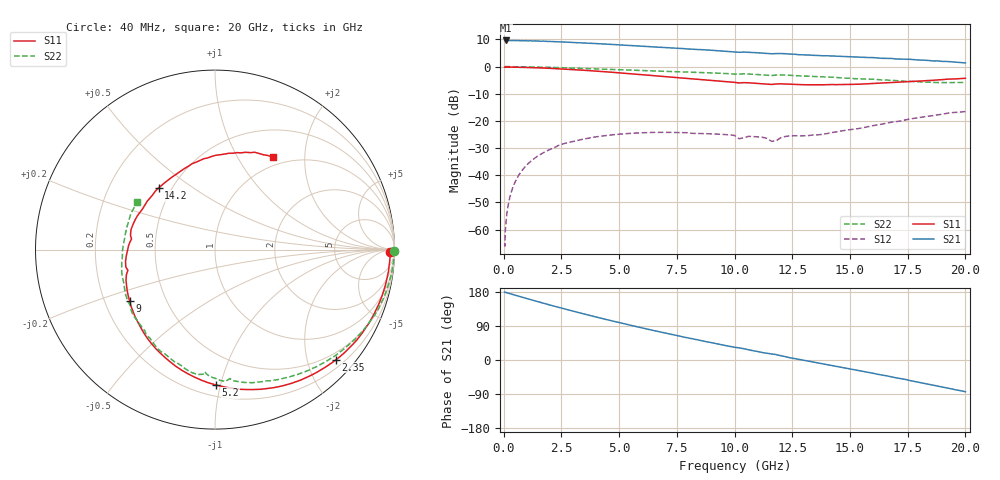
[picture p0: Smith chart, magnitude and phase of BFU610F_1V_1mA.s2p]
! Filename:  P:\Prog\Test\Noise\ATS_data\Testdata_Net\SplitFiles\BFU610_2W_A5_HighFreq_1V_1mA_D.s2p
! Date/Time: Wed 10/Aug/2011 16:54:31
! BFU610_2W_A5_HighFreq_1V_1mA_10mA_Bias1_R.s2p
! MDIF S-parameter v. bias file
! BFU610_2W_A5_HighFreq_1V_1mA_10mA
! Date/time Mon Aug 08 13:53:02 2011
! bias mode 1
! bias variable = I_out
! VAR bias_var= 1
! VAR V_out= 1.0002
! VAR I_out= 0.9900
! VAR V_in= 0.8512
! VAR I_in= 0.0075
! Device data file deembeded for feedlines and parallel
! Original file: \SplitFiles\BFU610_2W_A5_HighFreq_1V_1mA_R.s2p
! Feed-files: PR003V01_101208_Feed1.s2p, PR003V01_101208_Feed2.s2p
! Parallel-file: PR003V01_101208_Par.s2p
# MHz S MA R 50
!  Freq-MHz  S11-mag  S11-arg  S21-mag  S21-arg  S12-mag  S12-arg  S22-mag  S22-arg
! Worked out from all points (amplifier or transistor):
!   167 points, 40 MHz to 20 GHz, reference 50 ohm
!   highest |S21| = 9.6 dB at 80 MHz (marker M1)
!   |S21| within 3 dB of that: start of sweep to 7.784 GHz
!   unconditionally stable (mu >= 1): 7.808 GHz to end of sweep
!   at 550 MHz: K = 0.00, MSG = 25.6 dB, |S12| = -41.5 dB
!   at 4.2 GHz: K = 0.42, MSG = 17.0 dB, |S12| = -25.6 dB
!   at 20 GHz: K = 1.26, MAG = 5.9 dB, |S12| = -16.5 dB
!   S11 on the Smith chart (normalised r, x): 40 MHz: 66, -34; 2.35 GHz: 0.35, -2.54; 5.2 GHz: 0.28, -0.97; 9 GHz: 0.31, -0.26; 14.2 GHz: 0.42, +0.37; 20 GHz: 0.87, +1.43
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40  0.9764 -0.7  3.013 179.5  0.0005523 87.0  0.9971 -0.4
50  0.9721 -0.7  3.001 179.5  0.0004964 49.5  0.9974 -0.5
80  0.9759 -1.4  3.021 178.6  0.001091 91.6  0.9978 -0.8
140  0.9757 -2.5  3.008 177.5  0.002022 91.6  0.9976 -1.4
280  0.9746 -5.1  3.006 174.9  0.004164 90.3  0.9969 -2.9
650  0.9697 -11.9  2.995 168.4  0.009993 84.2  0.9934 -6.6
1350  0.9517 -24.5  2.967 156.2  0.02073 73.7  0.982 -13.6
2350  0.9117 -42.3  2.862 139.3  0.0351 60.9  0.9567 -23.3
3400  0.8587 -60.1  2.722 122.7  0.04579 46.8  0.9256 -32.7
4300  0.8074 -75.0  2.609 109.0  0.05292 36.8  0.8973 -40.2
5200  0.7544 -89.5  2.475 95.9  0.05794 27.8  0.8691 -47.4
6800  0.6626 -114.9  2.26 73.7  0.0616 13.6  0.8215 -59.7
7800  0.6108 -130.5  2.137 60.6  0.06112 6.7  0.7937 -67.0
9000  0.5555 -148.7  1.994 45.8  0.05772 1.4  0.7643 -75.9
10200  0.4987 -166.6  1.83 32.0  0.04702 -6.5  0.723 -83.4
11600  0.4688 172.8  1.719 16.0  0.04221 -1.2  0.6829 -94.6
12000  0.4813 166.6  1.736 11.4  0.04897 13.0  0.7027 -97.8
13400  0.4641 144.2  1.61 -5.2  0.05507 11.8  0.6571 -111.8
14200  0.4663 132.4  1.566 -14.2  0.06106 15.9  0.6379 -120.0
16800  0.5101 97.0  1.41 -44.6  0.09455 12.2  0.559 -152.6
18400  0.5537 77.4  1.294 -64.0  0.1223 1.6  0.5156 -179.2
20000  0.6087 57.9  1.167 -83.7  0.1488 -13.8  0.5097 148.5
